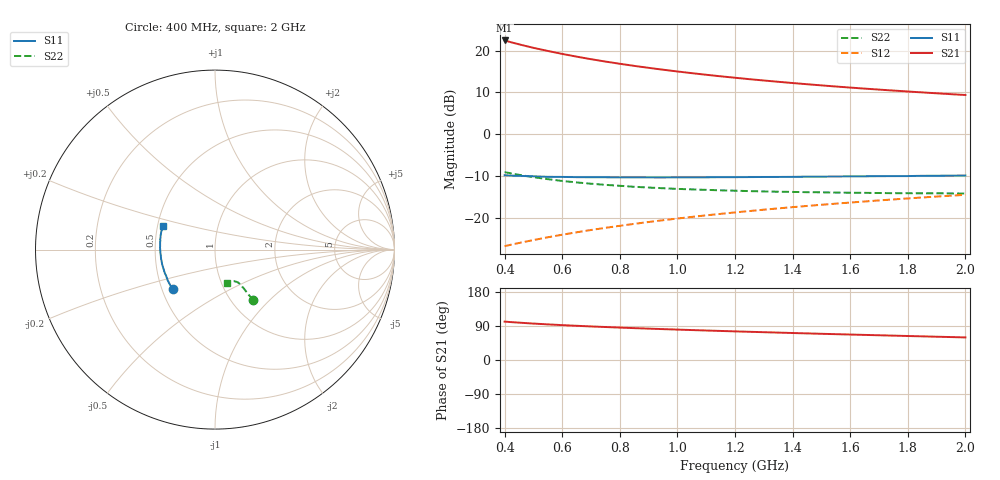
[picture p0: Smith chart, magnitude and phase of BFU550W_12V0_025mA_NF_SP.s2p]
! Filename:  P:\Prog\Test\Noise\ATS_data\Testdata_Net\06 Compressed Noise after Statistics\BFU550W_APM2013_11_D05_12p0V_025mA_NF_CM01_D.sf
! Date/Time: Tue 26/Mar/2013 16:25:26
! BFU550W_APM2013_11_D05_12p0V_1to35mA_NF_CM01_Bias8_R.sf
! Noise Parameter Data File
! BFU550W_APM2013_11_D05_12p0V_1to35mA_NF_CM01
! Date/time: Mon Mar 25 15:58:35 2013
! VAR V_out= 12.001000
! VAR I_out= 24.990000
! VAR V_in= 0.755000
! VAR I_in= 0.227400
! Device data file deembeded for feedlines and parallel
! Original file: \06 Compressed Noise after Statistics\BFU550W_APM2013_11_D05_12p0V_025mA_NF_CM01_R.sf
! Feed-files: PR019V01_070313_Feed1.s2p, PR019V01_070313_Feed2.s2p
! Parallel-file: PR019V01_070313_Par.s2p
# MHz S MA R 50
!  Freq-MHz  S11-mag  S11-arg  S21-mag  S21-arg  S12-mag  S12-arg  S22-mag  S22-arg
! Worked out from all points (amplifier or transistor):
!   37 points, 400 MHz to 2 GHz, reference 50 ohm
!   highest |S21| = 22.4 dB at 400 MHz (marker M1)
!   |S21| within 3 dB of that: start of sweep to 584.8 MHz
!   unconditionally stable (mu >= 1): 1.091 GHz to end of sweep
!   at 500 MHz: K = 0.89, MSG = 23.0 dB, |S12| = -25.3 dB
!   at 1.1 GHz: K = 1.00, MAG = 16.7 dB, |S12| = -19.4 dB
!   at 2 GHz: K = 1.01, MAG = 11.4 dB, |S12| = -14.5 dB
!   lowest NFmin = 1.11 dB at 420 MHz
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400  0.3227 -136.5  13.21 101.3  0.04586 66.5  0.352 -52.8
420  0.3208 -139.0  12.64 100.1  0.04754 66.8  0.3417 -53.0
440  0.3187 -141.2  12.12 99.1  0.0492 67.0  0.3315 -53.0
460  0.317 -143.2  11.64 98.1  0.05087 67.3  0.3225 -53.2
480  0.3152 -145.3  11.2 97.1  0.05257 67.5  0.3144 -53.3
500  0.3139 -147.3  10.78 96.2  0.05422 67.8  0.3065 -53.3
550  0.3092 -151.5  9.89 94.0  0.05855 68.4  0.29 -53.4
600  0.3086 -155.4  9.121 92.0  0.06284 68.8  0.276 -53.4
650  0.3065 -158.7  8.458 90.3  0.06719 69.2  0.2654 -53.5
700  0.3057 -161.9  7.886 88.6  0.07158 69.5  0.2559 -53.7
750  0.3056 -164.6  7.389 87.0  0.07594 69.7  0.248 -53.8
800  0.3043 -167.4  6.95 85.5  0.08032 69.8  0.2416 -54.2
850  0.3048 -169.9  6.561 84.1  0.08472 70.0  0.2352 -54.2
950  0.3038 -174.2  5.903 81.5  0.09367 70.0  0.2259 -54.9
1050  0.3048 -178.1  5.368 79.0  0.1026 70.0  0.219 -55.8
1150  0.3065 178.1  4.922 76.7  0.1116 69.8  0.2134 -56.8
1200  0.3064 176.6  4.731 75.5  0.1162 69.7  0.2112 -57.4
1350  0.3083 172.0  4.233 72.3  0.1297 69.1  0.2053 -59.1
1500  0.3108 167.6  3.834 69.2  0.1433 68.3  0.202 -61.5
1650  0.3139 163.6  3.508 66.2  0.1569 67.5  0.199 -63.9
1750  0.3156 161.4  3.325 64.3  0.166 66.9  0.1972 -65.7
2000  0.3214 155.4  2.942 59.6  0.1886 65.2  0.1956 -70.8
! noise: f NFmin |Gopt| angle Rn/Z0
400  1.125  0.2539  -173.5  0.0852
460  1.113  0.2599  -174.2  0.0871
600  1.141  0.2569  -170.8  0.0892
800  1.172  0.2859  -167.8  0.0812
1000  1.192  0.2907  -163.4  0.0838
1200  1.227  0.3054  -161.1  0.084
1400  1.272  0.321  -156.3  0.0825
1600  1.281  0.3275  -155.3  0.0876
1800  1.295  0.3443  -148.1  0.0946
2000  1.328  0.3635  -145.3  0.0976
